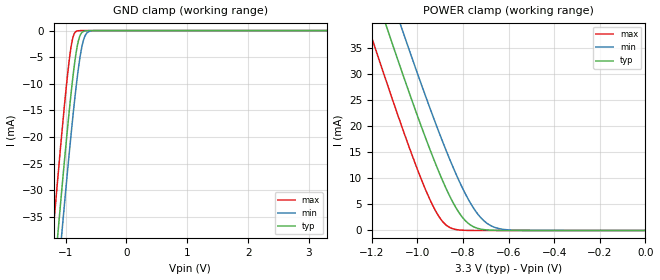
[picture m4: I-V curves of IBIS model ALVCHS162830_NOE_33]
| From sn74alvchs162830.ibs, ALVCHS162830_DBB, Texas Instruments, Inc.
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[Model]   ALVCHS162830_NOE_33
Model_type  Input
Vinl = 0.8
Vinh = 2.0
| variable   typ   min   max
C_comp   6.54pF   6.02pF   7.28pF
[Temperature Range]   40   100   -40
| Ambient temperature   25   85   -40
[Voltage range]   3.3   3   3.6
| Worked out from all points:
|   GND clamp passes 1 mA (typ) near -0.77 V on its own axis
|   POWER clamp passes 1 mA (typ) near -0.77 V on its own axis
[GND Clamp]
| ALVCHS162830_NOE_33
|   Voltage   I(typ)   I(min)   I(max)
-3.3V     -341.5mA   -348.9mA   -332.3mA
-1.215V   -49.6mA    -57.88mA   -38.96mA
-1.185V   -45.62mA   -53.91mA   -34.98mA
-1.125V   -37.77mA   -46.06mA   -27.13mA
-1.065V   -30.08mA   -38.33mA   -19.51mA
-920mV    -12.75mA   -20.53mA   -3.718mA
-875mV    -8.124mA   -15.45mA   -1.065mA
-825mV    -3.922mA   -10.26mA   -137.1uA
-775mV    -1.291mA   -5.83mA    -13.57uA
-715mV    -205.4uA   -2.128mA   -808.5nA
-585mV    -2.266uA   -70.82uA   -1.788nA
3.3V      6.304pA    16.45nA    5.63pA
[POWER Clamp]
| ALVCHS162830_NOE_33
|   Voltage   I(typ)   I(min)   I(max)
-3.3V     341.5mA    348.9mA    332.3mA
-1.24V    52.92mA    61.21mA    42.31mA
-1.2V     47.61mA    55.9mA     36.97mA
-1.125V   37.77mA    46.06mA    27.13mA
-1.065V   30.08mA    38.33mA    19.51mA
-960mV    17.26mA    25.26mA    7.377mA
-890mV    9.597mA    17.1mA     1.734mA
-795mV    2.124mA    7.484mA    34.55uA
-745mV    541.5uA    3.716mA    3.316uA
-700mV    123.8uA    1.543mA    399.1nA
-595mV    3.217uA    94.58uA    2.857nA
-48.03fV  6.304pA    8.354pA    6.677pA
